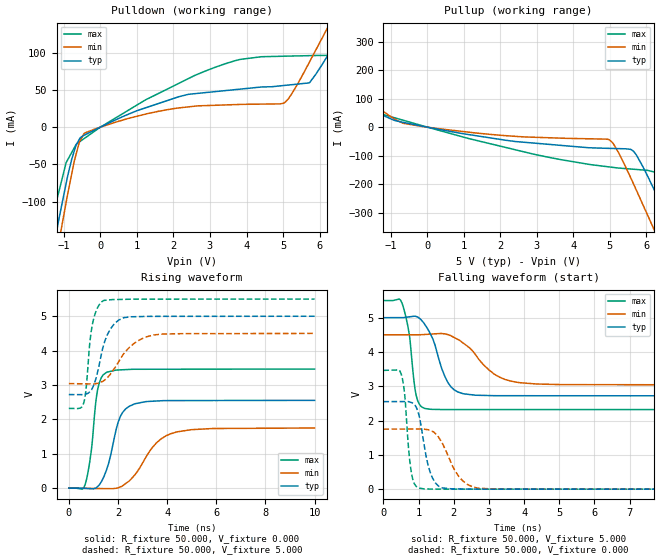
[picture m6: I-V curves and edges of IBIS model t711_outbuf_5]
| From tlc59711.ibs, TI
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|   t711_outbuf 5V Model
[Model] t711_outbuf_5
Model_type   Output
Polarity   Non-Inverting
Vmeas = 2.5
Vref = 2.6
Rref = 50
|   typ   min   max
|   (nom PVT)   (Fast PVT)   (slow PVT)
|   ON state : BUFFER OUTPUT TURNED HIGH
C_comp   1.98646E-12   1.61466E-12   2.27029E-12
|   OFF state: BUFFER OUTPUT TURNED LOW
|C_comp   1.92343E-12   1.92343E-12   1.92343E-12
| Where   nom PVT is  Nominal Process, 5V, 90C
|   Fast PVT is Strong Process, 4.5V, -40C
|   Slow PVT is Weak Process, 5.5V, 150C
|   C_comp - from L-C Tank method, L = 1nH, peak frequency
| variable   typ   min   max
[Voltage Range]   5   4.5   5.5
|Operating Temperature Range
|   25   85   -40
|Junction Temperature Range
[Temperature Range]   90   150   -40
[Pullup Reference]   5   4.5   5.5
[Pulldown Reference]   0   0   0
[Power Clamp Reference]   5   4.5   5.5
[GND Clamp Reference]   0   0   0
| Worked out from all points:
|   slope of the pulldown table from 0 to 0.75 V, typ, clamps not added: 44.2 ohm
|   slope of the pullup table from 0 to 0.75 V, typ, clamps not added: 42.1 ohm
|   falling waveform, R_fixture 50.000, V_fixture 5.000: 20-80 % time 472ps typ, 848ps min, 222ps max; typ from 5 V to 2.72 V
|   rising waveform, R_fixture 50.000, V_fixture 0.000: 20-80 % time 547ps typ, 1.06ns min, 315ps max; typ from 0 V to 2.55 V
|   rising waveform, R_fixture 50.000, V_fixture 5.000: 20-80 % time 528ps typ, 949ps min, 278ps max; typ from 2.72 V to 5 V
|   falling waveform, R_fixture 50.000, V_fixture 0.000: 20-80 % time 287ps typ, 520ps min, 163ps max; typ from 2.55 V to 0 V
[Pulldown]
|   Voltage   I(typ)   I(min)   I(max)
-5V       -1.198A    -1.28A     -1.081A
-1.59V    -246.7mA   -284.3mA   -184.7mA
-1.13V    -122mA     -153.2mA   -85.22mA
-667.9mV  -24.4mA    -37.01mA   -23.68mA
-425mV    -10.4mA    -7.838mA   -14.66mA
2.593V    44.92mA    28.14mA    69.55mA
5.015V    55.8mA     32.12mA    95.1mA
5.721V    59.34mA    87.09mA    95.88mA
6.236V    96.93mA    134.9mA    96.27mA
6.506V    119.4mA    161.1mA    104mA
7.559V    207.4mA    263.5mA    172.4mA
9.985V    423.5mA    510mA      347.6mA
[Pullup]
|   Voltage   I(typ)   I(min)   I(max)
-5V       352.5mA    416.3mA    271.4mA
-2.121V   114.8mA    142.1mA    82.14mA
-665.8mV  17.02mA    13.69mA    24.49mA
2.409V    -50.46mA   -32.32mA   -79.37mA
4.983V    -74.53mA   -44.47mA   -139.7mA
5.235V    -75.43mA   -89.33mA   -143.6mA
5.645V    -84.51mA   -198.8mA   -147.8mA
6.21V     -219.1mA   -359.7mA   -157.5mA
6.451V    -285.7mA   -430mA     -179.7mA
6.731V    -363.5mA   -511.9mA   -244.5mA
7.47V     -568.7mA   -727.8mA   -438.4mA
9.985V    -1.28A     -1.47A     -1.11A
[Ramp]
R_load = 50
|   typ   min   max
dV/dt_r   1.53194/5.45453e-010   1.04998/1.05314e-009   2.07826/3.12919e-010
dV/dt_f   1.40149/4.69699e-010  0.886365/8.37921e-010   1.90776/2.20636e-010
[Falling Waveform]
R_fixture = 50.000
V_fixture = 5.000
V_fixture_min = 4.500
V_fixture_max = 5.500
C_fixture = 0.000
|  time   V(typ)   V(min)   V(max)
0s        5V         4.5V       5.5V
530.2ps   5.001V     4.501V     5.422V
734.6ps   5.024V     4.501V     4.522V
930.4ps   5.034V     4.501V     2.744V
1.174ns   4.806V     4.511V     2.354V
1.834ns   3.11V      4.505V     2.321V
2.269ns   2.783V     4.26V      2.321V
3.145ns   2.726V     3.36V      2.321V
3.843ns   2.725V     3.11V      2.321V
10ns      2.722V     3.042V     2.32V
[Rising Waveform]
R_fixture = 50.000
V_fixture = 0.000
V_fixture_min = 0.000
V_fixture_max = 0.000
C_fixture = 0.000
|  time   V(typ)   V(min)   V(max)
0s        47.69uV    16.43uV    141uV
663ps     -6.8mV     -6.165mV   102.1mV
906.7ps   -16.73mV   -8.437mV   1.047V
1.169ns   43.84mV    -10.89mV   2.853V
1.551ns   568mV      -14.45mV   3.372V
2.08ns    2.059V     32.59mV    3.44V
2.677ns   2.451V     379.8mV    3.458V
3.558ns   2.534V     1.309V     3.459V
4.373ns   2.547V     1.631V     3.459V
10ns      2.553V     1.75V      3.464V
[Rising Waveform]
R_fixture = 50.000
V_fixture = 5.000
V_fixture_min = 4.500
V_fixture_max = 5.500
C_fixture = 0.000
|  time   V(typ)   V(min)   V(max)
0s        2.722V     3.042V     2.32V
602.3ps   2.719V     3.034V     2.468V
689.7ps   2.734V     3.033V     2.808V
843.1ps   2.797V     3.031V     4.141V
954.4ps   2.903V     3.03V      4.746V
1.413ns   4.154V     3.119V     5.456V
2.025ns   4.886V     3.671V     5.488V
2.699ns   4.987V     4.233V     5.497V
3.418ns   4.997V     4.451V     5.497V
10ns      5V         4.5V       5.5V
[Falling Waveform]
R_fixture = 50.000
V_fixture = 0.000
V_fixture_min = 0.000
V_fixture_max = 0.000
C_fixture = 0.000
|  time   V(typ)   V(min)   V(max)
0s        2.553V     1.75V      3.464V
509.5ps   2.554V     1.752V     3.346V
607.6ps   2.555V     1.752V     2.733V
785.9ps   2.529V     1.753V     547.9mV
1.013ns   2.15V      1.754V     31.43mV
1.323ns   512.2mV    1.715V     3.833mV
1.679ns   35.7mV     1.331V     722.7uV
2.156ns   6.561mV    353.3mV    690.4uV
2.689ns   1.291mV    28.67mV    654.2uV
10ns      79.15uV    40.84uV    158.5uV
